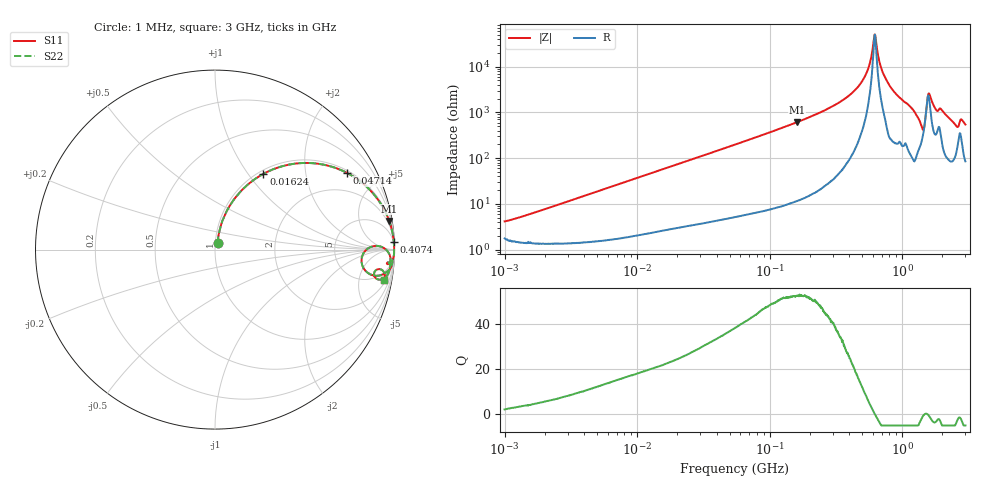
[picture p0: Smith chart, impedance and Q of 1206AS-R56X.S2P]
!s-Parameter Generated by FASTRON Sdn. Bhd.
!FASTRON P/N : 1206AS-R56X
!Keysight Technologies: E4991B_MY54100416_A.01.15
!Date created: Thu Nov 16 13:17:12 2023
!Version  : Rev00 Thu Nov 16 13:17:12 2023
!Data & Calibration Information:
!Freq	S11	S21	S12	S22
!PortZ  Port1:50+j0  Port2:50+j0
!When reading reference impedance value at option line is always used.
! Remarks : This data is being provided solely for informational purposes.
# Hz S dB R 50
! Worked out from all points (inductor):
!   1601 points, 1 MHz to 3 GHz, reference 50 ohm
!   read as one part in series: L = 598 nH near 1.203 MHz
!   highest Q = 52.8 at 160.6 MHz (marker M1), where L = 602 nH
!   self-resonance near 620.2 MHz
!   S11 on the Smith chart (normalised r, x): 1 MHz: 1.04, +0.08; 16.24 MHz: 1.05, +1.19; 47.14 MHz: 1.09, +3.40; 407.4 MHz: 3, +49; 3 GHz: 3, -11
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1000000  -27.79 62.7  -0.16 -2.1  -0.16 -2.1  -27.79 62.7
3804036  -17.11 76.3  -0.21 -8.0  -0.21 -8.0  -17.11 76.3
1.447069e7  -6.75 60.0  -1.24 -27.3  -1.24 -27.3  -6.75 60.0
1.623577e7  -6.01 57.4  -1.48 -30.0  -1.48 -30.0  -6.01 57.4
4.713729e7  -1.40 30.1  -6.00 -58.4  -6.00 -58.4  -1.40 30.1
5.477226e7  -1.08 26.5  -6.99 -62.0  -6.99 -62.0  -1.08 26.5
1.606197e8  -0.14 9.3  -15.82 -79.6  -15.82 -79.6  -0.14 9.3
2.083556e8  -0.08 6.9  -18.43 -82.0  -18.43 -82.0  -0.08 6.9
4.073935e8  -0.02 2.3  -27.89 -85.3  -27.89 -85.3  -0.02 2.3
5.311214e8  -0.02 0.9  -36.48 -82.4  -36.48 -82.4  -0.02 0.9
6.202446e8  -0.02 0.0  -54.06 -8.9  -54.06 -8.9  -0.02 0.0
6.993907e8  -0.02 -0.6  -38.86 78.5  -38.86 78.5  -0.02 -0.6
7.925923e8  -0.02 -1.4  -32.28 84.4  -32.28 84.4  -0.02 -1.4
1.243477e9  -0.12 -5.6  -20.17 79.5  -20.17 79.5  -0.12 -5.6
1.409185e9  -1.02 -9.2  -14.52 49.3  -14.52 49.3  -1.02 -9.2
1.45942e9  -1.73 -3.1  -14.54 13.7  -14.54 13.7  -1.73 -3.1
1.557514e9  -0.40 -0.2  -26.96 3.4  -26.96 3.4  -0.40 -0.2
1.604986e9  -0.25 -1.6  -28.25 42.9  -28.25 42.9  -0.25 -1.6
1.791767e9  -0.23 -4.6  -21.55 69.1  -21.55 69.1  -0.23 -4.6
2.530652e9  -0.48 -10.1  -14.93 67.4  -14.93 67.4  -0.48 -10.1
2.811057e9  -0.48 -7.4  -17.32 63.1  -17.32 63.1  -0.48 -7.4
3e9  -0.38 -10.1  -15.04 70.9  -15.04 70.9  -0.38 -10.1
